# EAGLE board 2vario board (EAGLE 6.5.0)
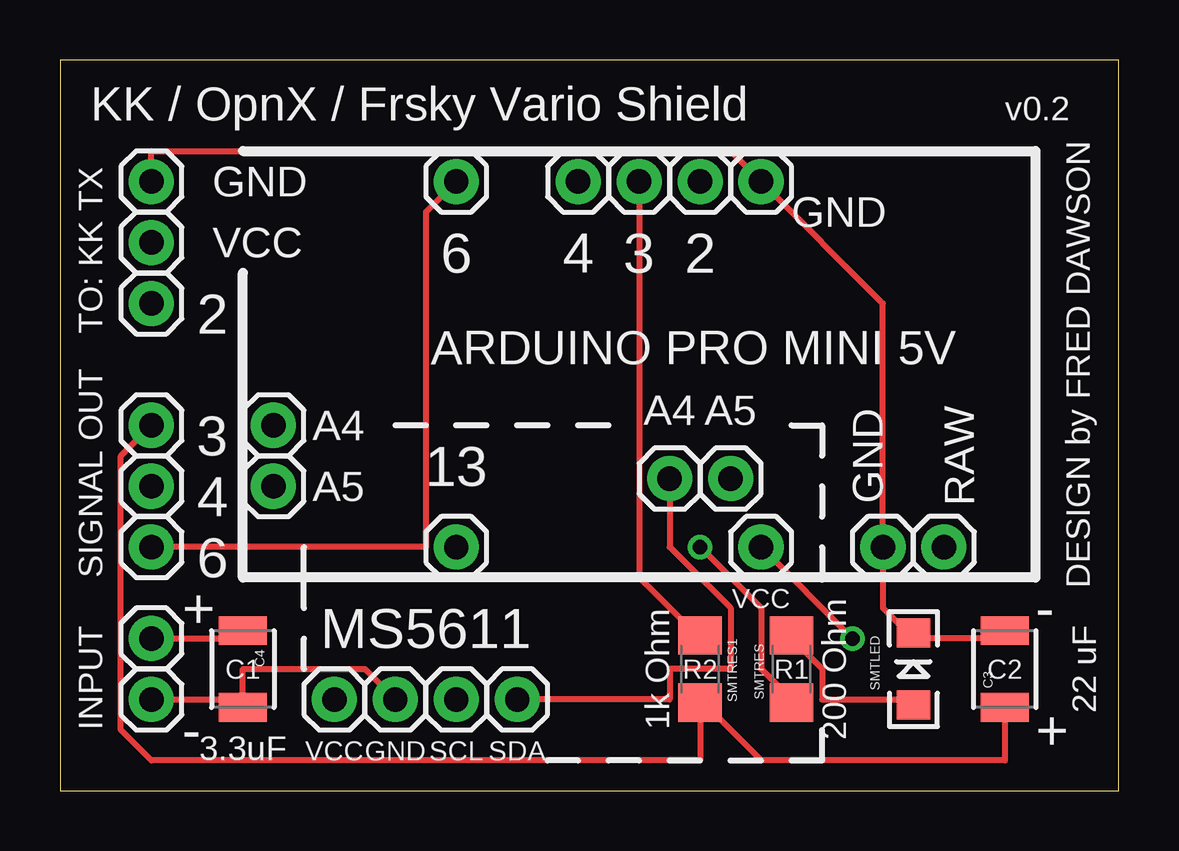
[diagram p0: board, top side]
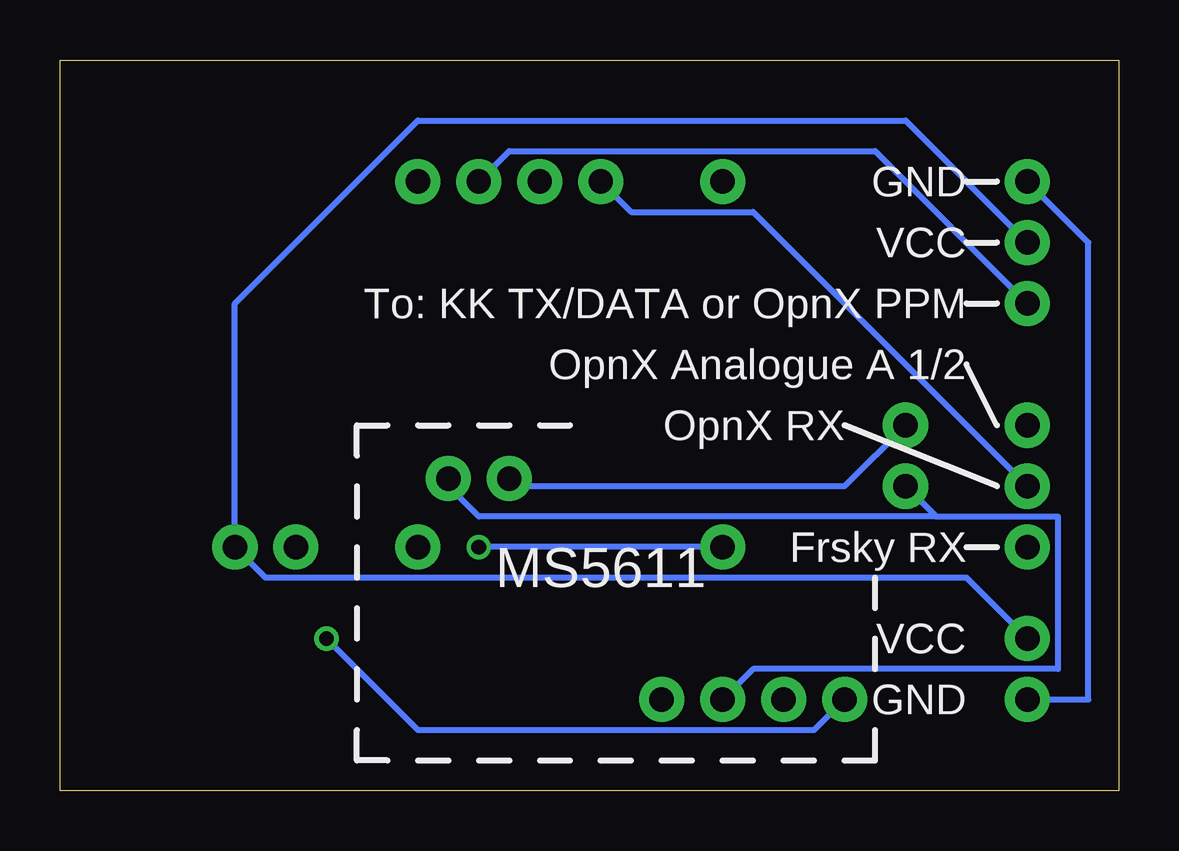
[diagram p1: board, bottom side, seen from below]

Size 44.12 x 30.47 mm. Coordinates in mm from the lower left corner, seen from the top.
Outline: 0,0 44.12,0 44.12,30.47 0,30.47 0,0
Copper layers (1*16): Top 0.035mm / dielectric 1.5mm / Bottom 0.035mm
Design rules "default": minimum track width 10mil, minimum drill 24mil, track to track 8mil, track to pad 8mil, pad to pad 8mil, via to via 8mil, smd to smd 8mil, copper to edge 40mil, drill to drill 8mil, minimum pad ring 10mil, minimum via ring 8mil, stop-mask expansion 4mil, vias tented up to drill 0mil, thermal gap 10mil

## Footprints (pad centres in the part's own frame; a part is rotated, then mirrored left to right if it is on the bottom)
1210 = smd 1.2 x 2: 1 -1.6,0; 2 1.6,0
1X01 = drill 1.016 pad 1.88: 1 0,0
LED-1206 = smd 1.2 x 1.4: A -1.5,0; C 1.5,0
1206 = smd 1.6 x 1.8: 1 -1.4,0; 2 1.4,0

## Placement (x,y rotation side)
C3  10uF  [1210]  39.37,5.08 90 top
C4  10uF  [1210]  7.62,5.08 270 top
JP1  M01PTH  [1X01]  11.43,3.81 0 top
JP2  M01PTH  [1X01]  16.51,25.4 0 top
JP3  M01PTH  [1X01]  29.21,10.16 0 top
JP4  M01PTH  [1X01]  13.97,3.81 0 top
JP5  M01PTH  [1X01]  16.51,3.81 0 top
JP6  M01PTH  [1X01]  19.05,3.81 0 top
JP7  M01PTH  [1X01]  3.81,22.86 0 top
JP8  M01PTH  [1X01]  16.51,10.16 0 top
JP9  M01PTH  [1X01]  8.89,15.24 0 top
JP10  M01PTH  [1X01]  8.89,12.7 0 top
JP11  M01PTH  [1X01]  27.94,13.02 0 top
JP12  M01PTH  [1X01]  25.4,13.02 0 top
JP13  M01PTH  [1X01]  3.81,6.35 0 top
JP14  M01PTH  [1X01]  3.81,3.81 0 top
JP15  M01PTH  [1X01]  3.81,20.32 0 top
JP16  M01PTH  [1X01]  3.81,25.4 0 top
JP17  M01PTH  [1X01]  36.83,10.16 0 top
JP18  M01PTH  [1X01]  3.81,10.16 0 top
JP19  M01PTH  [1X01]  34.29,10.16 0 top
JP20  M01PTH  [1X01]  26.67,25.4 0 top
JP21  M01PTH  [1X01]  24.13,25.4 0 top
JP22  M01PTH  [1X01]  21.59,25.4 0 top
JP23  M01PTH  [1X01]  3.81,12.7 0 top
JP24  M01PTH  [1X01]  3.81,15.24 0 top
JP25  M01PTH  [1X01]  29.21,25.4 0 top
SMTLED  [LED-1206]  35.56,5.08 90 top
SMTRES  [1206]  30.48,5.08 90 top
SMTRES1  [1206]  26.67,5.08 270 top

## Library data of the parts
C3 C4 = SparkFun-Capacitors; PROD_ID: CAP-09824
JP1-JP25 = SparkFun-Connectors
SMTLED = SparkFun-LED
SMTRES SMTRES1 = SparkFun-Resistors

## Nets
GND: C3.2 C4.2 JP4.1 JP14.1 JP16.1 JP19.1 JP25.1 SMTLED.C
N$1: C3.1 JP24.1 SMTRES1.2
N$2: SMTLED.A SMTRES.2
N$3: JP8.1 SMTRES.1
N$4: JP15.1 JP20.1
N$5: JP1.1 JP3.1
N$6: JP2.1 JP18.1
N$7: JP6.1 JP9.1 JP12.1
N$8: JP5.1 JP10.1 JP11.1
N$9: JP22.1 JP23.1
N$10: JP21.1 SMTRES1.1
V+: C4.1 JP7.1 JP13.1 JP17.1

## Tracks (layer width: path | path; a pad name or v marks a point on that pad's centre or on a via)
GND
  Top 0.254: 35.56,6.35 39.37,6.35 C3.2 | 35.56,6.35 34.29,7.62 JP19.1 34.29,20.32 JP25.1 27.94,26.67 3.81,26.67 JP16.1 | 35.56,6.35 SMTLED.C | JP14.1 7.62,3.81 | JP4.1 12.7,5.08 7.62,5.08 7.62,3.81 | 7.62,3.81 C4.2
  Bottom 0.254: JP16.1 1.27,22.86 1.27,3.81 JP14.1
N$1
  Top 0.254: 39.37,3.81 C3.1 39.37,1.27 29.21,1.27 26.67,3.81 SMTRES1.2 26.67,1.27 3.81,1.27 2.54,2.54 2.54,13.97 JP24.1
N$2
  Top 0.254: SMTLED.A 35.56,3.81 31.75,3.81 31.75,5.08 30.48,6.35 SMTRES.2
N$3  (via drill 0.61)
  Top 0.254: v26.67,10.16 29.21,7.62 29.21,5.08 30.48,3.81 SMTRES.1
  Bottom 0.254: JP8.1 v26.67,10.16
N$4
  Bottom 0.254: JP15.1 10.16,26.67 25.4,26.67 JP20.1
N$5  (via drill 0.61)
  Top 0.254: JP3.1 v33.02,6.35
  Bottom 0.254: JP1.1 12.7,2.54 29.21,2.54 v33.02,6.35
N$6
  Top 0.254: JP18.1 15.24,10.16 15.24,24.13 JP2.1
N$7
  Top 0.254: JP6.1 25.4,3.81 25.4,5.08 27.94,5.08 27.94,7.62 25.4,10.16 JP12.1
  Bottom 0.254: JP9.1 11.43,12.7 25.4,12.7 JP12.1
N$8
  Bottom 0.254: JP5.1 15.24,5.08 2.54,5.08 2.54,11.43 7.62,11.43 | JP10.1 7.62,11.43 | 7.62,11.43 26.67,11.43 27.94,12.7 JP11.1
N$9
  Bottom 0.254: JP23.1 15.24,24.13 20.32,24.13 JP22.1
N$10
  Top 0.254: JP21.1 24.13,8.89 26.67,6.35 SMTRES1.1
V+
  Top 0.254: JP13.1 7.62,6.35 C4.1
  Bottom 0.254: JP7.1 8.89,27.94 29.21,27.94 36.83,20.32 JP17.1 35.56,8.89 6.35,8.89 JP13.1

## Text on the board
tPlace: KK / OpnX / Frsky Vario Shield | v0.2 | GND | GND | VCC | 6 | 4 | 3 | 2 | TO: KK TX | 2 | ARDUINO PRO MINI 5V | DESIGN by FRED DAWSON | A4 | A4 | A5 | 3 | GND | RAW | A5 | 13 | 4 | SIGNAL OUT | 6 | + | MS5611 | VCC | - | C1 | 1k Ohm | R2 | R1 | 200 Ohm | C2 | 22 uF | INPUT | - | + | 3.3uF | VCC | GND | SCL | SDA
bPlace: GND | VCC | To: KK TX/DATA or OpnX PPM | OpnX Analogue A 1/2 | OpnX RX | Frsky RX | MS5611 | VCC | GND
